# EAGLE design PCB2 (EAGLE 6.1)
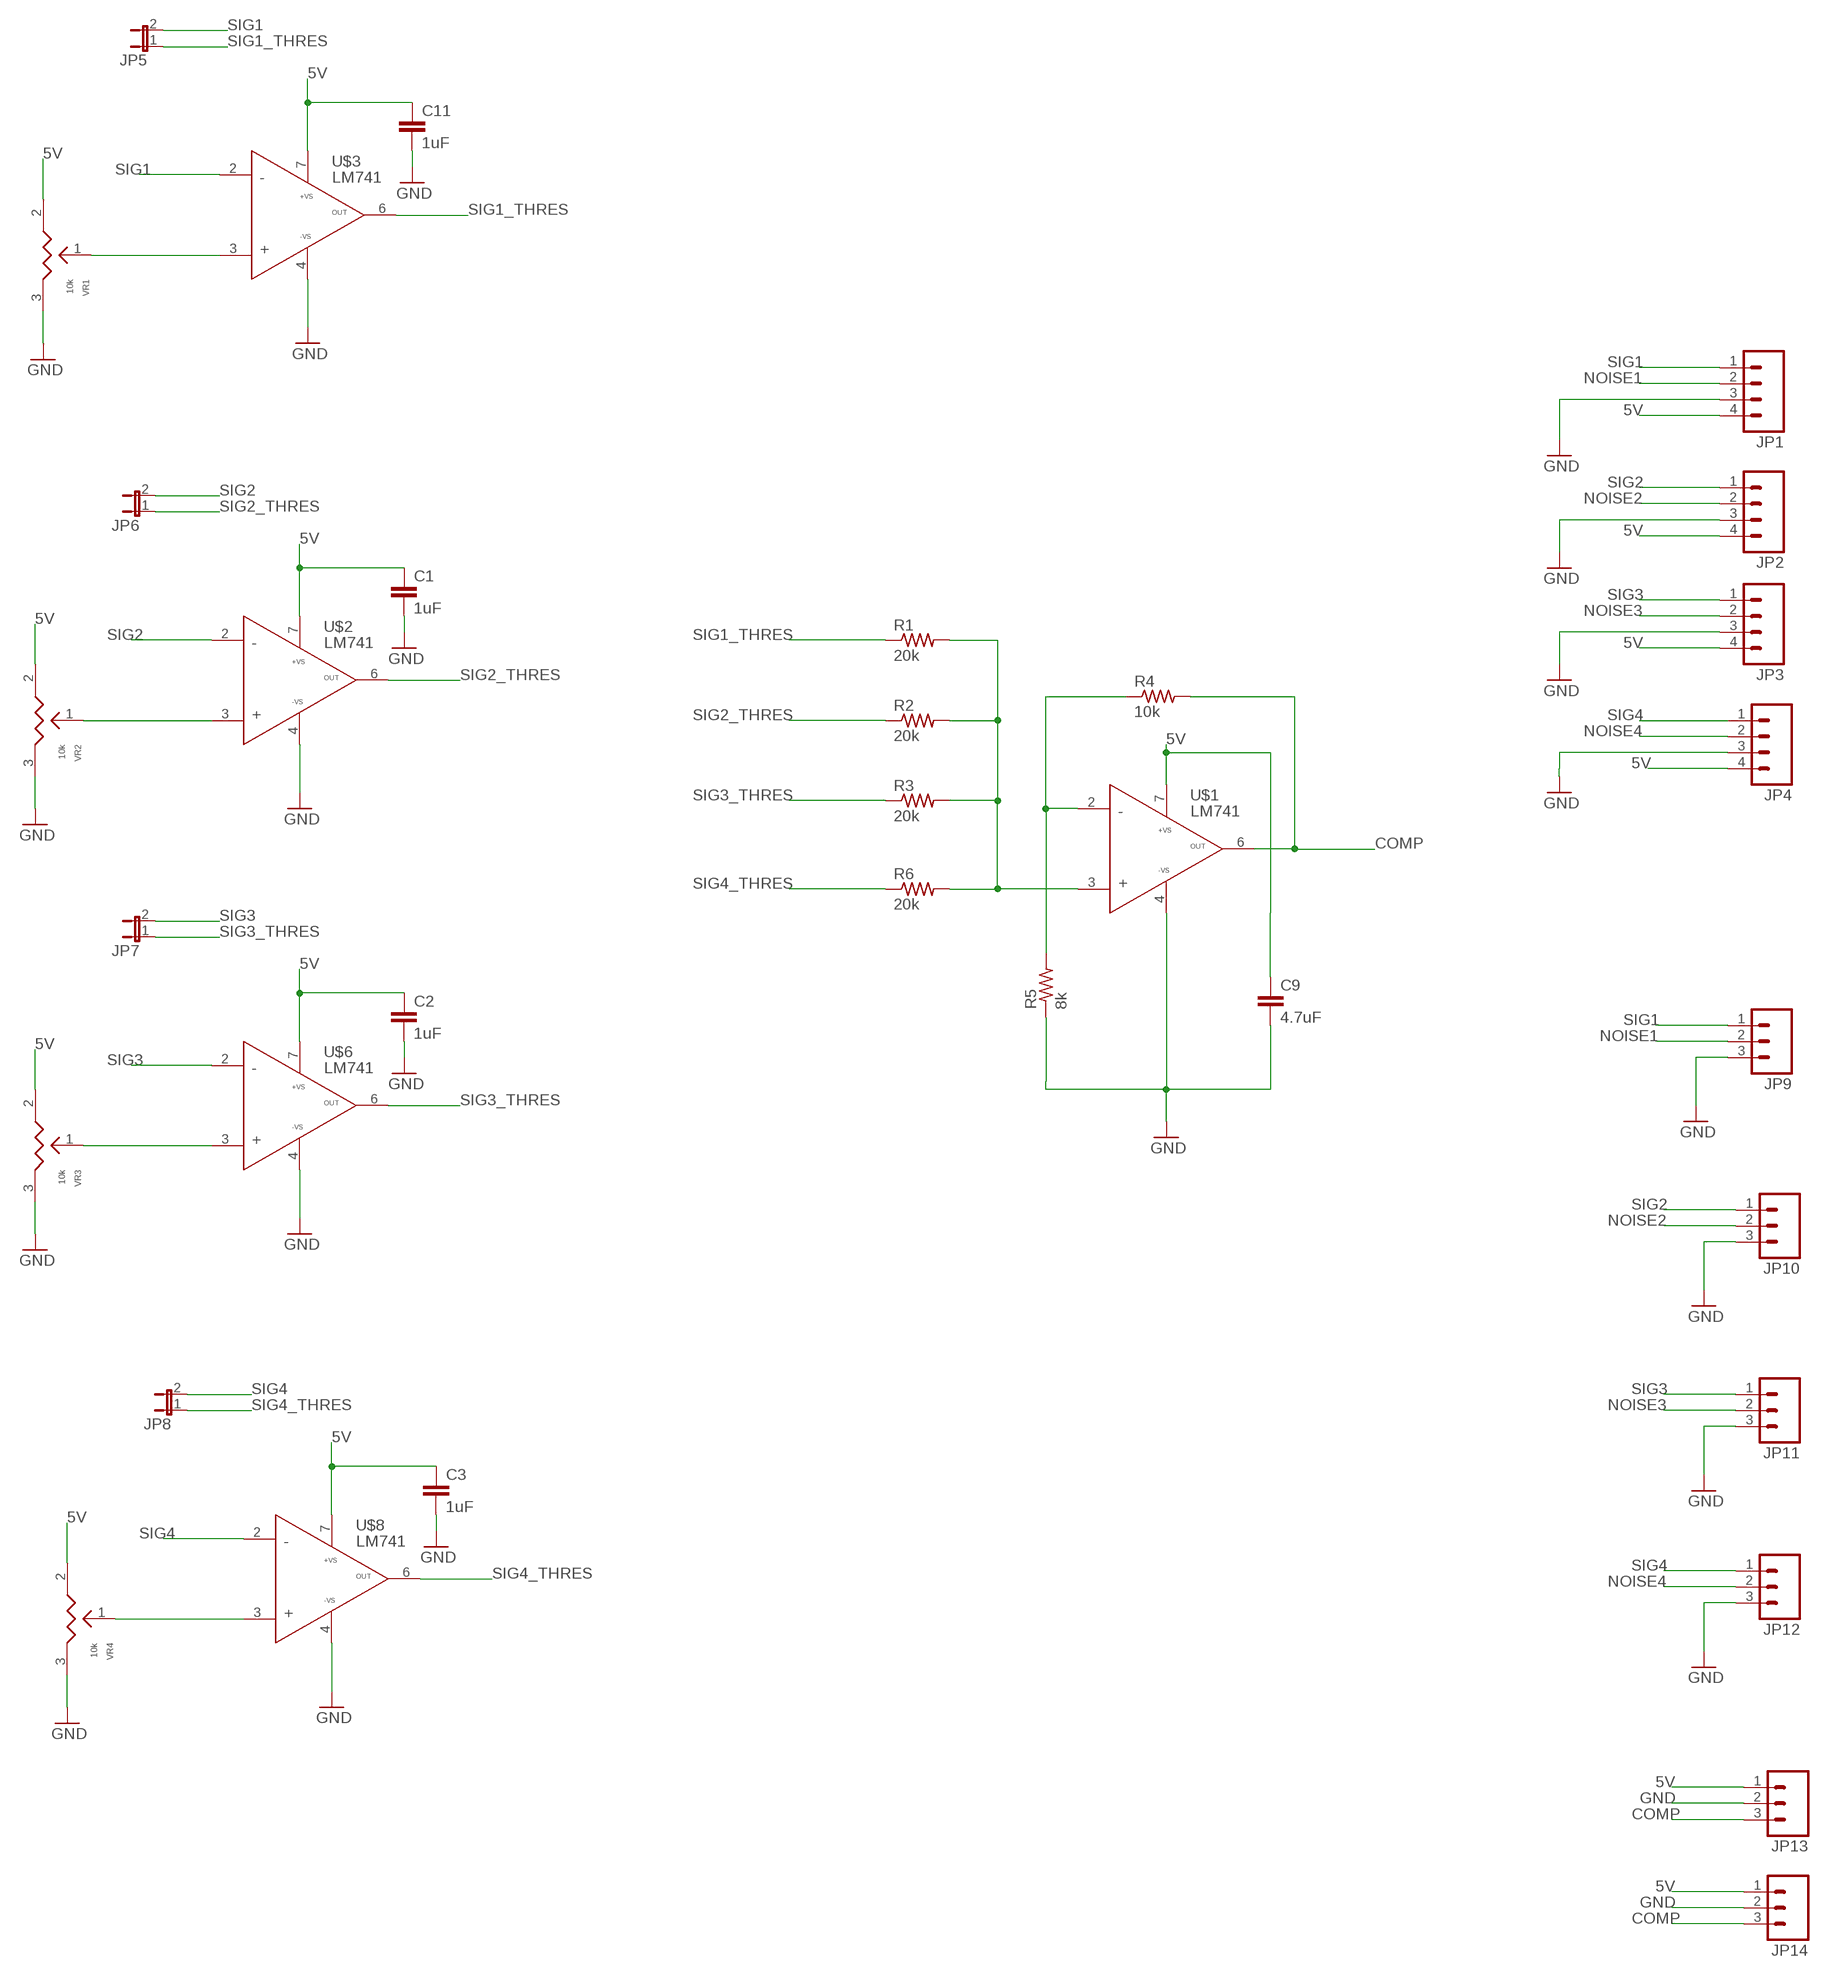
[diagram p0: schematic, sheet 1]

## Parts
C1  1uF  C-EUC1206  [C1206]
C2  1uF  C-EUC1206  [C1206]
C3  1uF  C-EUC1206  [C1206]
C9  4.7uF  C-EUC1206  [C1206]
C11  1uF  C-EUC1206  [C1206]
JP1  M04PTH  [1X04]
JP2  M04PTH  [1X04]
JP3  M04PTH  [1X04]
JP4  M04PTH  [1X04]
JP5  JP1E  [JP1]
JP6  JP1E  [JP1]
JP7  JP1E  [JP1]
JP8  JP1E  [JP1]
JP9  M03PTH  [1X03]
JP10  M03PTH  [1X03]
JP11  M03PTH  [1X03]
JP12  M03PTH  [1X03]
JP13  M03PTH  [1X03]
JP14  M03PTH  [1X03]
R1  20k  R-US_R1206  [R1206]
R2  20k  R-US_R1206  [R1206]
R3  20k  R-US_R1206  [R1206]
R4  10k  R-US_R1206  [R1206]
R5  8k  R-US_R1206  [R1206]
R6  20k  R-US_R1206  [R1206]
U$1  LM741  [DIP08]
U$2  LM741  [DIP08]
U$3  LM741  [DIP08]
U$6  LM741  [DIP08]
U$8  LM741  [DIP08]
VR1  10k  POTENTIO_METER-3386H  [3386H]
VR2  10k  POTENTIO_METER-3386H  [3386H]
VR3  10k  POTENTIO_METER-3386H  [3386H]
VR4  10k  POTENTIO_METER-3386H  [3386H]

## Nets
5V: C1.1 C2.1 C3.1 C9.1 C11.1 JP1.4 JP2.4 JP3.4 JP4.4 JP13.1 JP14.1 U$1.7 U$2.7 U$3.7 U$6.7 U$8.7 VR1.2 VR2.2 VR3.2 VR4.2
COMP: JP13.3 JP14.3 R4.2 U$1.6
GND: C1.2 C2.2 C3.2 C9.2 C11.2 JP1.3 JP2.3 JP3.3 JP4.3 JP9.3 JP10.3 JP11.3 JP12.3 JP13.2 JP14.2 R5.1 U$1.4 U$2.4 U$3.4 U$6.4 U$8.4 VR1.3 VR2.3 VR3.3 VR4.3
N$1: R1.2 R2.2 R3.2 R6.2 U$1.3
N$2: R4.1 R5.2 U$1.2
N$3: U$6.3 VR3.1
N$4: U$3.3 VR1.1
N$5: U$2.3 VR2.1
N$6: U$8.3 VR4.1
NOISE1: JP1.2 JP9.2
NOISE2: JP2.2 JP10.2
NOISE3: JP3.2 JP11.2
NOISE4: JP4.2 JP12.2
SIG1: JP1.1 JP5.2 JP9.1 U$3.2
SIG1_THRES: JP5.1 R1.1 U$3.6
SIG2: JP2.1 JP6.2 JP10.1 U$2.2
SIG2_THRES: JP6.1 R2.1 U$2.6
SIG3: JP3.1 JP7.2 JP11.1 U$6.2
SIG3_THRES: JP7.1 R3.1 U$6.6
SIG4: JP4.1 JP8.2 JP12.1 U$8.2
SIG4_THRES: JP8.1 R6.1 U$8.6

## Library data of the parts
C1-C3 C9 C11 = resistor:C-EU: CAPACITOR, European symbol
JP1-JP4 = SparkFun-Connectors:M04: Header 4 Standard 4-pin 0.1" header. Use with straight break away headers (SKU : PRT-00116), right angle break away headers (PRT-00553), swiss pins (PRT-00743), machine pins (PRT-00117), and female headers (PRT-00115). Molex polarized connector foot print use with SKU : PRT-08231 with associated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
JP5-JP8 = jumper:JP1E: JUMPER
JP9-JP14 = SparkFun-Connectors:M03: Header 3 Standard 3-pin 0.1" header. Use with straight break away headers (SKU : PRT-00116), right angle break away headers (PRT-00553), swiss pins (PRT-00743), machine pins (PRT-00117), and female headers (PRT-00115). Molex polarized connector foot print use with SKU : PRT-08232 with associated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
R1-R6 = resistor:R-US_: RESISTOR, American symbol
U$1-U$3 U$6 U$8 = LM741:LM741: OPAMP
VR1-VR4 = POT-3386H:POTENTIO_METER-3386H

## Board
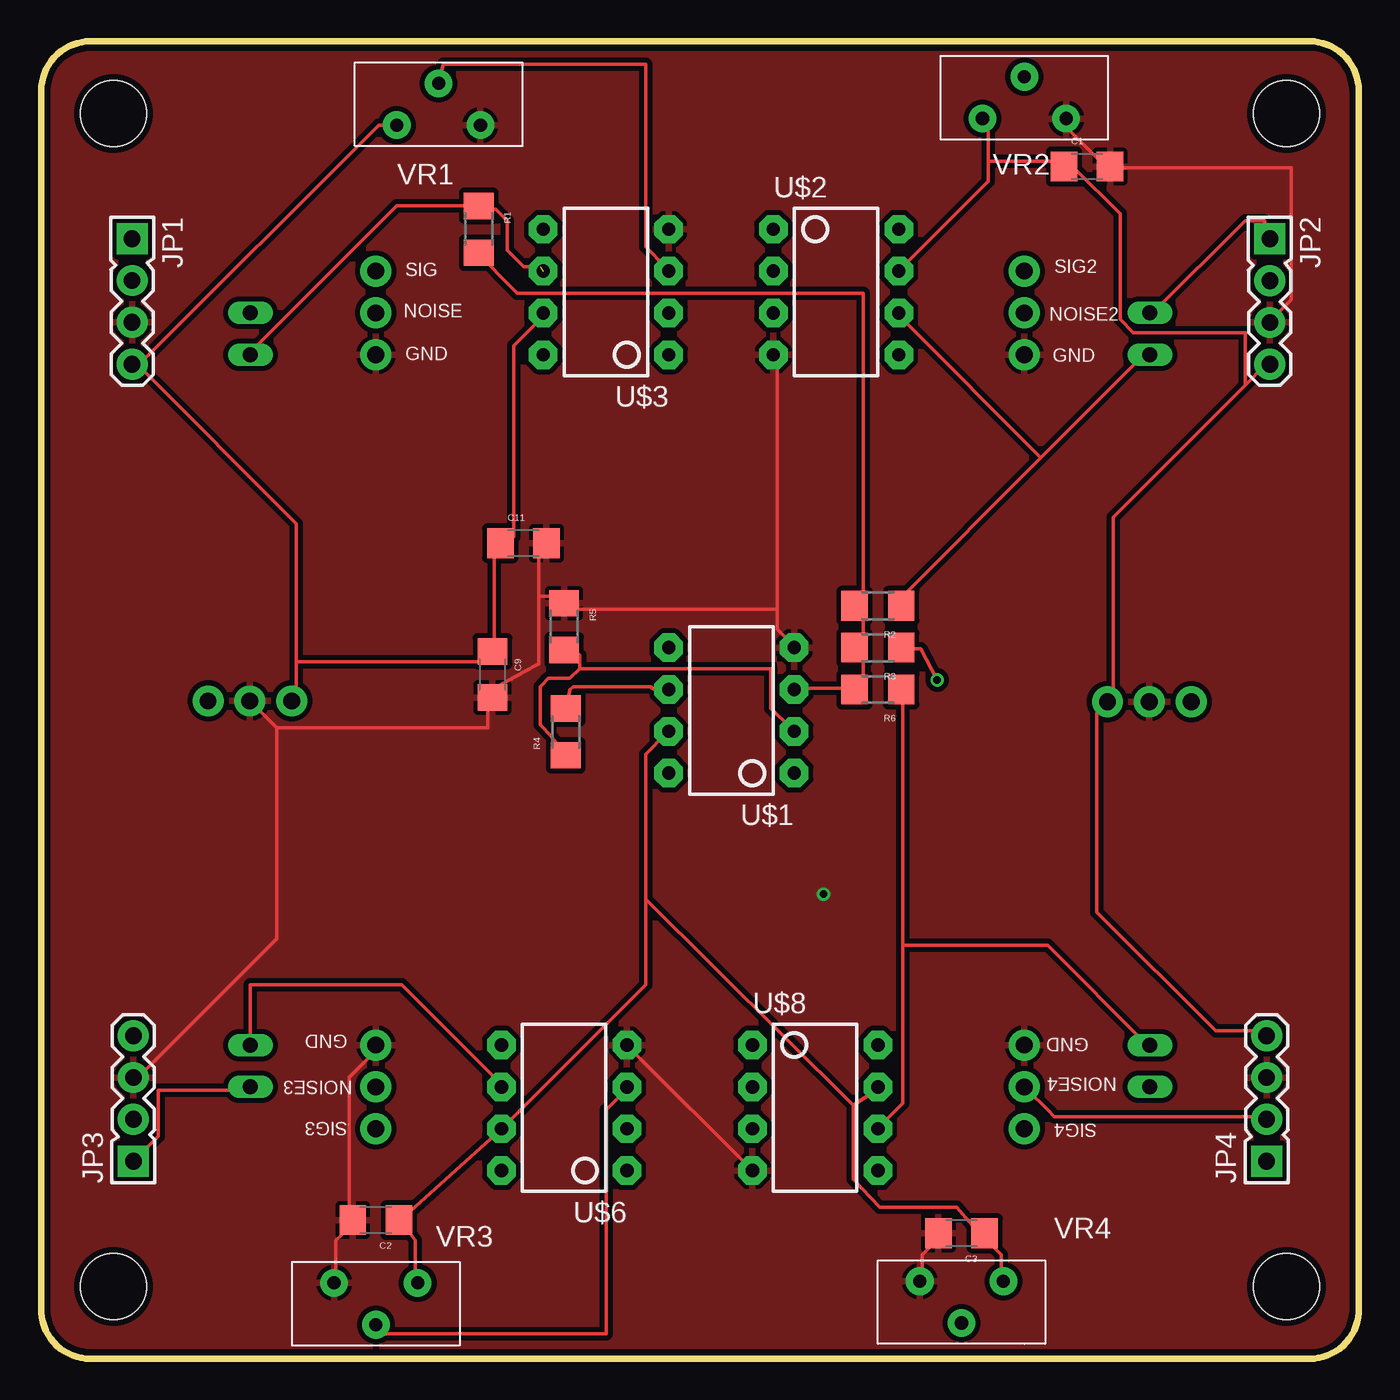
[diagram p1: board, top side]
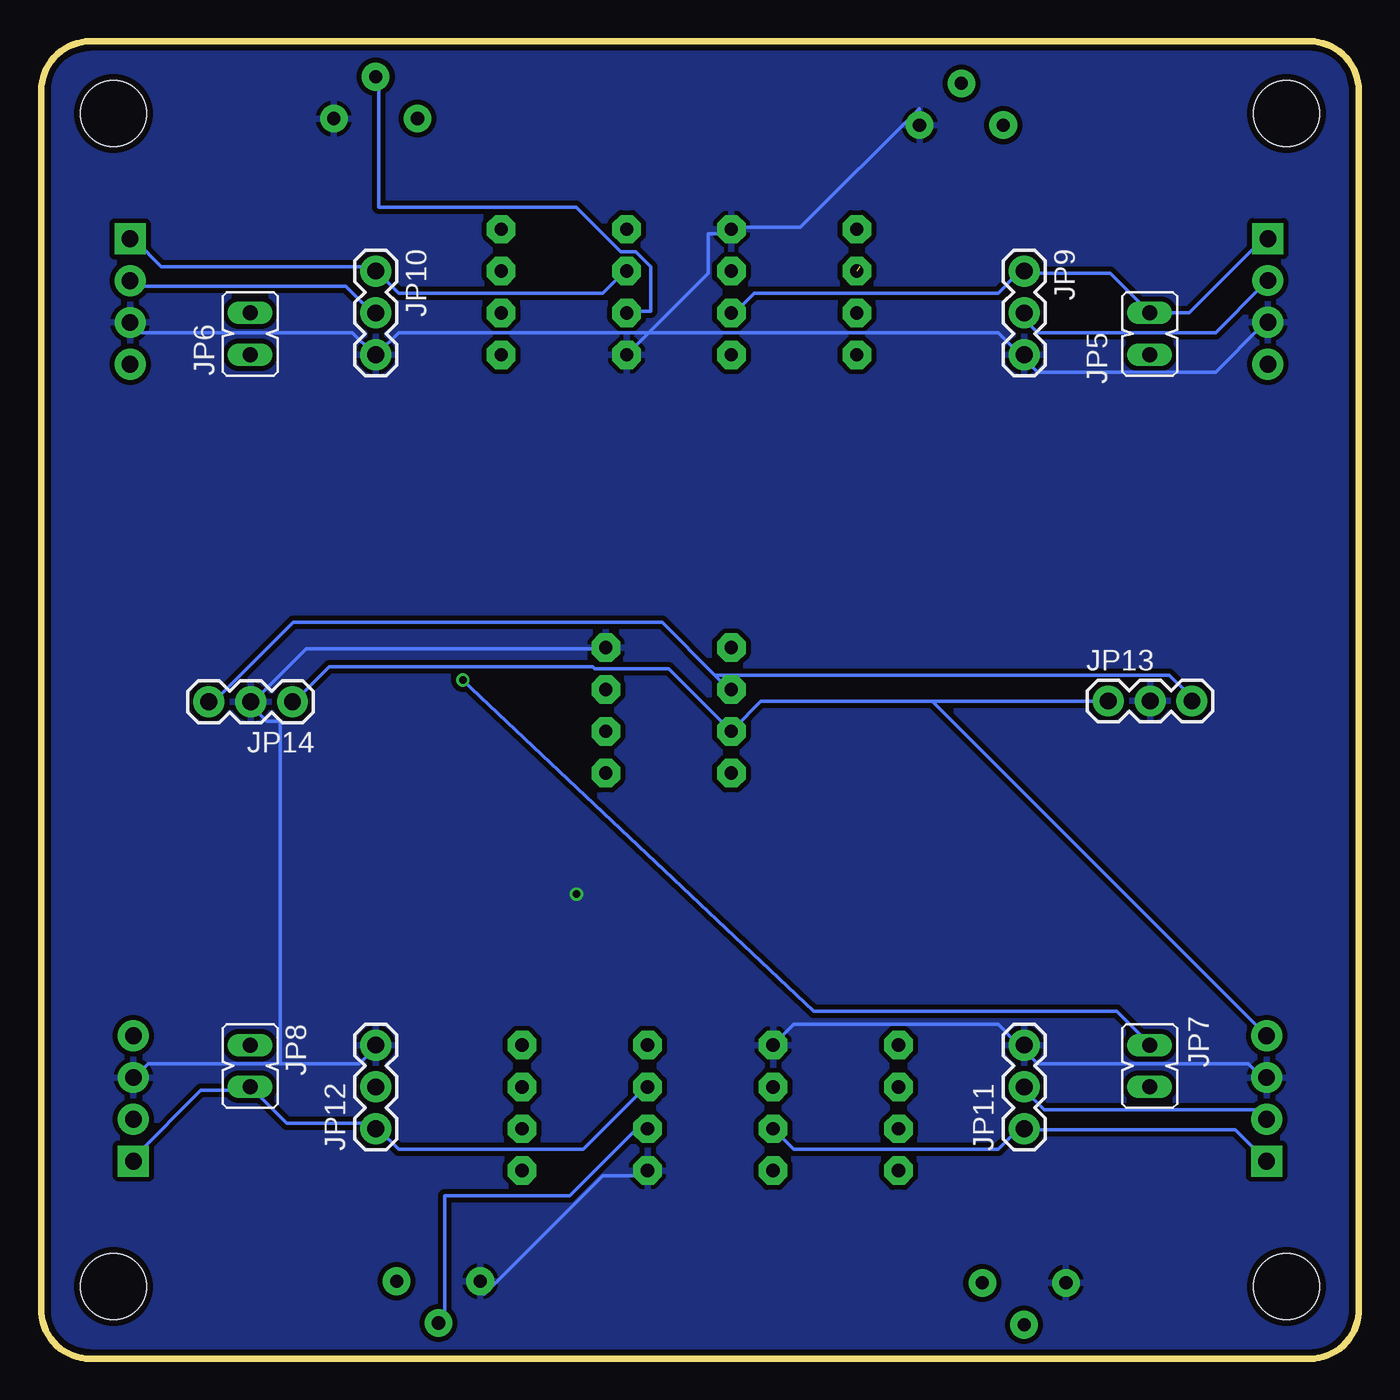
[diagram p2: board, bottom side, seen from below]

Size 80 x 80 mm. Coordinates in mm from the lower left corner, seen from the top.
Outline: 3,0 77,0
Outline: 77,0 3,0
Outline: 3,0 arc-86 0,2.8 0,77 arc-90 3,80 77,80 arc-90 80,77 80,2.8 arc-86 77,0
Copper layers (1*16): Top 0.0356mm / dielectric 1.5011mm / Bottom 0.0356mm
Design rules: minimum track width 6mil, minimum drill 13mil, track to track 6mil, track to pad 6mil, pad to pad 6mil, via to via 6mil, smd to smd 6mil, copper to edge 15mil, drill to drill 6mil, minimum pad ring 7mil, minimum via ring 7mil, stop-mask expansion 3mil, vias tented up to drill 0mil, thermal gap 10mil
Holes 4 mm at 75.6,4.4 4.4,4.4 4.4,75.6 75.6,75.6

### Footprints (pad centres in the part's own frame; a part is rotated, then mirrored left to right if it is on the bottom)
C1206 = smd 1.6 x 1.8: 1 -1.4,0; 2 1.4,0
1X04 = drill 1.016 pad 1.88 square: 1 0,0 | drill 1.016 pad 1.88: 2 2.54,0; 3 5.08,0; 4 7.62,0
JP1 = drill 0.914 long: 1 0,-1.27; 2 0,1.27
1X03 = drill 1.016 pad 1.88: 1 0,0; 2 2.54,0; 3 5.08,0
R1206 = smd 1.6 x 1.803: 1 -1.422,0; 2 1.422,0
DIP08 = drill 0.813 pad 1.727 octagon: 1 -3.81,-3.81; 2 -1.27,-3.81; 3 1.27,-3.81; 4 3.81,-3.81; 5 3.81,3.81; 6 1.27,3.81; 7 -1.27,3.81; 8 -3.81,3.81
3386H = drill 0.8 pad 1.676: 1 2.54,2.54; 2 0,0; 3 5.08,0

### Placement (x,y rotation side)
C1  63.5,72.39 0 top
C2  20.32,8.42 180 top
C3  55.88,7.62 180 top
C9  27.4,41.55 270 top
C11  29.28,49.52 0 top
JP1  5.52,68.01 270 top
JP2  74.6,68 270 top
JP3  5.6,12 90 top
JP4  74.4,12 90 top
JP5  12.7,62.23 0 bottom
JP6  67.31,62.23 0 bottom
JP7  12.7,17.78 180 bottom
JP8  67.31,17.78 180 bottom
JP9  20.32,66.04 270 bottom
JP10  59.69,66.04 270 bottom
JP11  20.32,13.97 90 bottom
JP12  59.69,13.97 90 bottom
JP13  15.21,39.94 0 bottom
JP14  64.74,39.89 180 bottom
R1  26.57,68.58 270 top
R2  50.8,45.72 180 top
R3  50.8,43.18 180 top
R4  31.85,38.07 90 top
R5  31.75,44.45 270 top
R6  50.8,40.64 180 top
U$1  41.91,39.37 90 top
U$2  48.26,64.77 270 top
U$3  34.29,64.77 90 top
U$6  31.75,15.24 90 top
U$8  46.99,15.24 270 top
VR1  21.59,74.9 0 top
VR2  57.15,75.3 0 top
VR3  22.86,4.61 180 top
VR4  58.42,4.71 180 top

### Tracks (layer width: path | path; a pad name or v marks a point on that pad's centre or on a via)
5V
  Top 0.2: 57.5,72.71 62.3,72.71 C1.1 62.7,72.31 65.5,69.51 65.5,63.11 66.3,62.31 73.1,62.31 73.1,59.11 | 57.5,72.71 57.5,74.91 VR2.2 | 57.5,72.71 57.5,71.51 52.3,66.31 U$2.7 | JP4.4 74.3,19.91 71.3,19.91 64.1,27.11 64.1,39.21 64.8,39.91 64.78,39.89 JP14.1 65.08,39.89 65.1,39.91 65.1,51.11 65.25,51.26 73.1,59.11 | 73.1,59.11 74.3,60.31 JP2.4 | 5.9,60.31 20.5,74.91 VR1.2 | 5.9,60.31 JP1.4 5.9,60.31 | U$3.7 30.3,63.11 28.7,61.51 28.7,49.91 C11.1 28.3,49.51 27.5,48.71 27.5,42.71 C9.1 27.1,42.31 15.5,42.31 | VR4.2 58.3,4.91 58.3,6.31 57.1,7.51 C3.1 56.7,7.91 55.6,9.21 50.9,9.21 49.3,10.91 49.3,15.41 | 49.3,15.41 50.7,16.31 U$8.7 | 21.8,8.41 22.7,7.21 22.7,4.71 VR3.2 | 21.8,8.41 C2.1 21.8,8.41 | 21.8,8.41 27.9,13.91 U$6.7 28.3,14.31 36.7,22.71 36.7,27.91 | 36.7,27.91 36.7,36.71 37.9,37.91 U$1.7 | 36.7,27.91 49.3,15.41 | 15.5,42.31 15.5,40.31 15.5,40.23 JP13.1 | 5.9,60.31 15.5,50.71 15.5,42.31
  Bottom 0.2: 25.9,39.91 15.5,39.91 15.24,39.91 JP13.1 | 25.9,39.91 36.3,39.91 37.9,38.31 U$1.7 38.3,38.31 41.75,41.76 41.9,41.91 46.4,41.91 46.5,42.01 62.5,42.01 64.6,39.91 JP14.1 | 25.9,39.91 5.9,19.91 JP3.4
COMP
  Top 0.2: 31.5,39.91 R4.2 32.1,40.57 32.1,40.61 32.3,40.81 35.8,40.81 36.99,40.81 37.28,40.62 U$1.6
  Bottom 0.2: 39.1,41.51 38.3,40.71 U$1.6 | 39.1,41.51 42.3,44.71 64.7,44.71 69.45,39.96 69.5,39.91 69.52,39.89 JP14.3 | 39.1,41.51 11.5,41.51 10.3,40.31 10.3,39.94 JP13.3
GND  (via drill 0.45)
  Top 0.2: 18.9,8.11 17.9,7.21 17.9,3.91 VR3.3 | 18.9,8.11 C2.2 19.1,7.91 18.9,8.11 | 18.9,8.11 18.7,8.31 18.7,17.11 20.3,18.71 JP11.3 | C3.2 54.7,7.51 53.5,6.31 53.5,3.91 VR4.3 | U$6.4 35.9,18.71 43.1,11.51 U$8.4 | 30.2,46.31 31.5,46.31 31.5,45.51 R5.1 31.9,45.51 44.7,45.51 | 30.2,46.31 30.2,48.71 C11.2 | 30.2,46.31 30.2,42.21 27.5,40.71 C9.2 27.1,40.31 27.1,38.31 14.3,38.31 | 14.3,38.31 12.7,39.91 12.67,39.91 JP13.2 | VR2.3 62.3,75.91 62.3,74.71 64.3,72.71 C1.2 64.7,72.31 75.9,72.31 75.9,64.31 74.7,63.11 JP2.3 | 44.7,45.51 44.7,60.71 U$2.4 | 44.7,45.51 44.7,44.31 45.5,43.51 U$1.4 | 14.3,38.31 14.3,25.51 5.9,17.11 JP3.3
  Bottom 0.2: JP3.3 5.9,17.11 6.7,17.91 19.5,17.91 20.3,18.71 JP11.3 20.7,19.11 21.9,20.31 34.3,20.31 35.5,19.11 U$6.4 | VR4.3 53.1,3.91 45.9,11.11 43.5,11.11 U$8.4 | JP1.3 5.9,62.71 8.7,59.91 19.5,59.91 20.3,60.71 JP9.3 20.7,61.11 21.9,62.31 43.1,62.31 | 65.5,17.91 73.5,17.91 74.3,17.11 JP4.3 | 65.5,17.91 60.7,17.91 59.9,18.71 JP12.3 | VR1.3 26.7,75.91 33.9,68.71 37.9,68.71 U$3.4 38.3,68.31 39.5,68.31 39.5,65.91 43.1,62.31 | 43.1,62.31 44.3,61.11 U$2.4 | 43.1,62.31 58.3,62.31 59.5,61.11 JP10.3 59.9,61.11 61.1,62.31 73.9,62.31 74.3,62.71 JP2.3 | 67.1,39.91 63.9,43.11 45.9,43.11 U$1.4 | 65.5,17.91 65.5,38.71 66.3,38.71 67.1,39.51
  other vias: 47.5,28.21
  pour Top (isolate 0.305): 3,79.81 77,79.81 arc-90 80,76.81 80,2.71 arc-90 77.1,-0.19 3,-0.19 arc-90 0,2.81 0,76.91 arc-90 2.9,79.81
  pour Bottom (isolate 0.305): 3,80.01 77,80.01 arc-90 80,77.01 80,2.91 arc-90 77.1,0.01 3,0.01 arc-90 0,3.01 0,77.11 arc-90 2.9,80.01
N$1
  Top 0.2: 49.9,40.71 49.9,43.11 R3.2 49.9,43.51 49.9,45.51 R2.2 49.9,45.91 49.9,64.71 28.9,64.71 28.7,64.91 26.5,67.11 26.55,67.16 R1.2 | 49.9,40.71 R6.2 49.9,40.71 | 49.9,40.71 45.9,40.71 U$1.3
N$2
  Top 0.2: 32.7,41.91 32.7,42.71 31.9,43.51 R5.2 | 32.7,41.91 44.3,41.91 44.3,39.51 45.5,38.31 U$1.2 | 32.7,41.91 32.1,41.31 30.8,41.31 30.4,40.91 30.3,40.81 30.3,38.51 30.4,38.41 arc-11 R4.1
N$3
  Top 0.2: VR3.1 20.7,1.51 34.3,1.51 34.3,15.11 35.5,16.31 U$6.3
N$4
  Top 0.2: VR1.1 24.4,78.61 36.7,78.61 36.7,67.51 37.9,66.31 U$3.3
N$5
  Bottom 0.2: VR2.1 59.5,77.71 59.5,69.91 47.5,69.91 44.8,67.21 43.9,67.21 43,66.31 43,63.61 44.2,63.61 U$2.3
N$6
  Bottom 0.2: VR4.1 55.5,1.51 55.5,9.91 47.9,9.91 43.9,13.91 43.5,13.91 U$8.3
NOISE1
  Bottom 0.2: JP9.2 20.3,63.11 19.5,62.31 8.7,62.31 5.9,65.11 JP1.2
NOISE2
  Bottom 0.2: JP10.2 59.9,63.51 61.5,65.11 74.3,65.11 JP2.2
NOISE3
  Bottom 0.2: JP3.2 5.9,14.71 6.3,15.11 19.1,15.11 20.3,16.31 JP11.2
NOISE4
  Top 0.2: JP4.2 74.3,14.71 61.5,14.71 61.1,15.11 59.9,16.31 JP12.2
SIG1
  Bottom 0.2: JP5.2 15.1,65.91 20.3,65.91 JP9.1 20.7,65.91 21.9,64.71 36.7,64.71 37.9,63.51 U$3.2 | JP5.2 | JP5.2 10.3,63.51 5.9,67.91 JP1.1
SIG1_THRES  (1 unrouted)
  Top 0.2: JP5.1 12.7,61.11 19.1,67.51 21.59,70 R1.1 26.76,69.81 27.6,69.81 28.3,69.11 28.3,67.31 29.3,66.31 30.3,66.31
SIG2
  Top 0.2: JP6.2 67.5,63.51 73.1,69.11 74.3,69.11 74.3,68.31 JP2.1
  Bottom 0.2: U$2.2 44.7,65.91 45.9,64.71 58.3,64.71 59.5,65.91 JP10.1 59.9,66.31 72.7,66.31 74.3,67.91 JP2.1
SIG2_THRES
  Top 0.2: 60.7,54.71 67.1,61.11 JP6.1 | 60.7,54.71 51.9,45.91 R2.1 | 60.7,54.71 52.3,63.11 U$2.6
SIG3
  Top 0.2: JP7.2 12.7,16.31 7.1,16.31 7.1,13.51 5.9,12.31 JP3.1
  Bottom 0.2: U$6.2 35.5,13.91 34.3,12.71 21.9,12.71 20.7,13.91 JP11.1 20.3,13.91 7.5,13.91 5.9,12.31 JP3.1
SIG3_THRES  (via drill 0.45)
  Top 0.2: v54.4,41.21 53.4,43.11 51.9,43.11 R3.1 | U$6.6 27.9,16.71 21.9,22.71 12.7,22.71 12.7,19.11 JP7.1
  Bottom 0.2: v54.4,41.21 33.1,21.11 14.7,21.11 12.7,19.11 JP7.1
SIG4
  Bottom 0.2: U$8.2 43.5,16.31 47.1,12.71 58.3,12.71 59.5,13.91 JP12.1 59.9,14.31 65.1,14.31 67.1,16.31 JP8.2 67.5,16.31 70.3,16.31 74.3,12.31 JP4.1
SIG4_THRES
  Top 0.2: 52.3,25.11 52.3,15.51 51.1,14.31 U$8.6 | 52.3,25.11 52.3,39.91 51.9,40.31 R6.1 | 52.3,25.11 61.1,25.11 67.1,19.11 JP8.1

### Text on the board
tPlace: SIG | SIG2 | NOISE | NOISE2 | GND | GND | GND | GND | NOISE3 | NOISE4 | SIG3 | SIG4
